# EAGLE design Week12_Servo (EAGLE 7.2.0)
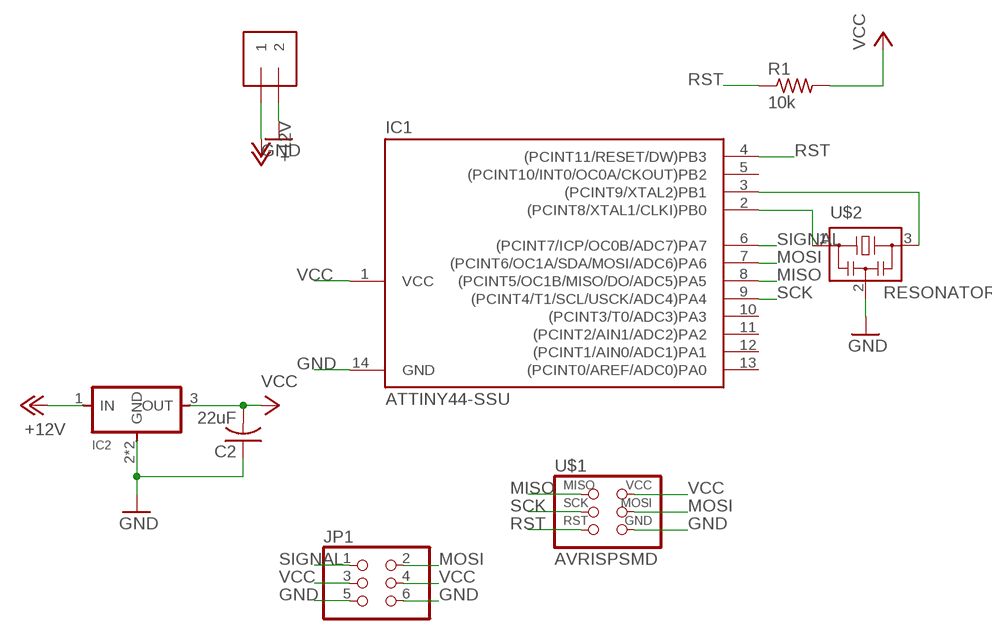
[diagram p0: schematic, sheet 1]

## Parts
C2  22uF  C-USC1206  [C1206]
IC1  ATTINY44-SSU  [SOIC14]
IC2  REGULATORSOT223  [SOT223]
J1  1X2-3.5MM  [3.5MMTERM]
JP1  PINHD-2X3-SMD  [2X03SMD]
R1  10k  RESISTOR1206  [1206]
U$1  AVRISPSMD  [2X03SMD]
U$2  RESONATOR  [EFOBM]

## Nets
+12V: IC2.1(IN) J1.1
GND: C2.1 IC1.14(GND) IC2.2(GND) IC2.4(GND) J1.2 JP1.5 JP1.6 U$1.6(GND) U$2.2
MISO: IC1.8((PCINT5/OC1B/MISO/DO/ADC5)PA5) U$1.1(MISO)
MOSI: IC1.7((PCINT6/OC1A/SDA/MOSI/ADC6)PA6) JP1.2 U$1.4(MOSI)
N$1: IC1.3((PCINT9/XTAL2)PB1) U$2.3
N$2: IC1.2((PCINT8/XTAL1/CLKI)PB0) U$2.1
RST: IC1.4((PCINT11/RESET/DW)PB3) R1.1 U$1.5(RST)
SCK: IC1.9((PCINT4/T1/SCL/USCK/ADC4)PA4) U$1.3(SCK)
SIGNAL: IC1.6((PCINT7/ICP/OC0B/ADC7)PA7) JP1.1
VCC: C2.2 IC1.1(VCC) IC2.3(OUT) JP1.3 JP1.4 R1.2 U$1.2(VCC)
Unconnected: IC1.5((PCINT10/INT0/OC0A/CKOUT)PB2) IC1.10((PCINT3/T0/ADC3)PA3) IC1.11((PCINT2/AIN1/ADC2)PA2) IC1.12((PCINT1/AIN0/ADC1)PA1) IC1.13((PCINT0/AREF/ADC0)PA0)

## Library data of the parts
C2 = 01_adafruit:C-US: CAPACITOR, American symbol
IC1 = 01_FAB_Hello:ATTINY44
IC2 = 01_fab:REGULATOR
J1 = 01_adafruit:1X2: 3.5mm Terminal block
JP1 = 01_FAB_Hello:PINHD-2X3-SMD: PIN HEADER
R1 = 01_FAB_Hello:RESISTOR
U$1 = 01_FAB_Hello:AVRISP
U$2 = 01_fab:RESONATOR

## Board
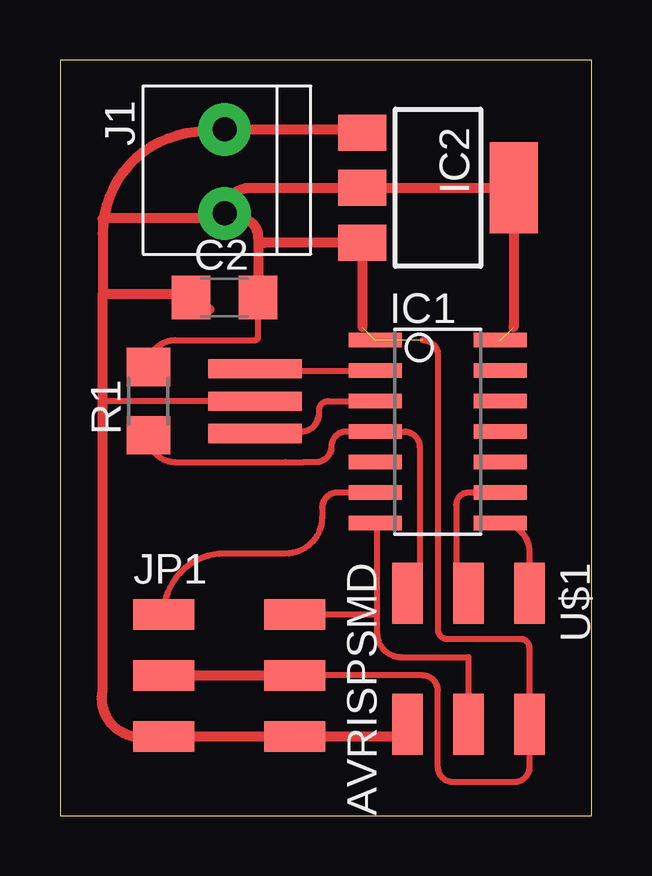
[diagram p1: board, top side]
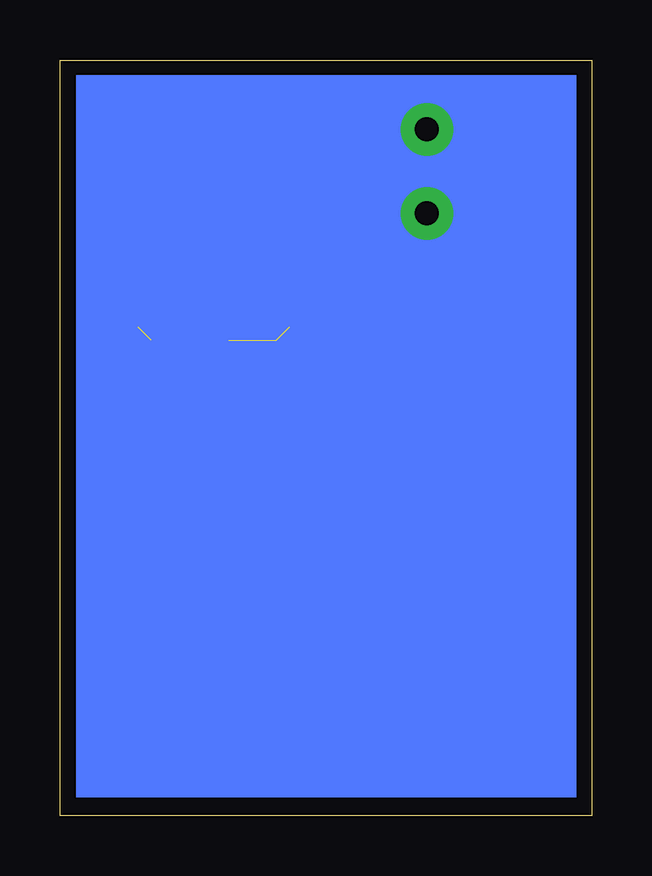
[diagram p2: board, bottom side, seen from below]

Size 22.15 x 31.49 mm. Coordinates in mm from the lower left corner, seen from the top.
Outline: 0,0 22.15,0 22.15,31.49 0,31.49 0,0
Copper layers (1*16): Top 0.035mm / dielectric 1.5mm / Bottom 0.035mm
Design rules "fabmodule": minimum track width 10mil, minimum drill 0.4mm, track to track 0.42mm, track to pad 0.42mm, pad to pad 0.42mm, via to via 0.42mm, smd to smd 0.42mm, copper to edge 40mil, drill to drill 0.8mm, minimum pad ring 10mil, minimum via ring 8mil, stop-mask expansion 4mil, vias tented up to drill 0mil, thermal gap 10mil

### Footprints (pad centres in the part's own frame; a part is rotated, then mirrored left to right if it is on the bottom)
C1206 = smd 1.6 x 1.8: 1 -1.4,0; 2 1.4,0
SOIC14 = smd 0.61 x 2.21: 1 -3.81,-2.603; 2 -2.54,-2.603; 3 -1.27,-2.603; 4 0,-2.603; 5 1.27,-2.603; 6 2.54,-2.603; 7 3.81,-2.603; 8 3.81,2.603; 9 2.54,2.603; 10 1.27,2.603; 11 0,2.603; 12 -1.27,2.603; 13 -2.54,2.603; 14 -3.81,2.603
SOT223 = smd 1.5 x 2: 1 -2.3,-3.15; 2 0,-3.15; 3 2.3,-3.15 | smd 3.8 x 2: 4 0,3.15
3.5MMTERM = drill 1 pad 2.184: 1 1.8,0; 2 -1.7,0
2X03SMD = smd 2.54 x 1.27: 1 -2.54,2.54; 2 2.92,2.54; 3 -2.54,0; 4 2.92,0; 5 -2.54,-2.54; 6 2.92,-2.54
1206 = smd 1.6 x 1.803: 1 -1.422,0; 2 1.422,0
EFOBM = smd 0.8 x 3.9: 1 -1.35,0; 2 0,0; 3 1.35,0

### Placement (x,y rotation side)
C2  6.86,21.59 0 top
IC1  15.75,16 270 top
IC2  15.75,26.16 270 top
J1  6.86,26.8 90 top
JP1  6.86,5.84 0 top
R1  3.68,17.27 90 top
U$1  17.02,6.73 270 top
U$2  8.13,17.27 270 top

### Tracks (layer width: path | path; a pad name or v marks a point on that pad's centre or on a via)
+12V
  Top 0.406: J1.1 12.6,28.6 IC2.1
GND  (1 unrouted)
  Top 0.254: U$2.2 1.78,17.27
  Top 0.406: U$1.6 14.48,3.56 arc-90 14.22,3.3 JP1.6 JP1.5 3.05,3.3 arc-90 1.78,5.21 1.78,17.27 1.78,21.72 | 18.9,20.36 IC2.4 IC2.2 7.92,26.16 arc90 J1.2 arc-90 6.65,24.89 1.78,24.89 1.78,24.26 | 6.22,21.08 C2.1 arc90 5.33,21.72 1.78,21.72 | 6.02,28.5 arc90 1.78,24.26 | 1.78,24.26 1.78,21.72
MISO
  Top 0.254: IC1.8 arc-90 19.56,10.98 U$1.1
MOSI
  Top 0.254: IC1.7 arc-90 13.21,12.13 13.21,8.38 | 13.21,8.38 13.21,7.62 arc90 14.22,6.6 17.02,6.6 U$1.4 | JP1.2 13.21,8.38
N$1
  Top 0.254: U$2.3 arc-90 8.21,16 10.03,16 arc90 10.79,16.76 10.79,16.89 arc-90 11.18,17.27 IC1.3
N$2
  Top 0.254: U$2.1 arc90 8.21,18.54 IC1.2
RST
  Top 0.254: U$1.5 arc90 14.86,9.65 arc90 14.99,9.78 14.99,15.37 arc90 14.35,16 IC1.4 11.94,16 arc90 11.3,15.37 arc-90 10.67,14.73 10.16,14.73 9.4,14.73 4.8,14.73 arc-90 R1.1
  Top 0.406: 14.86,10.03 14.73,10.03 arc90 14.48,9.78 U$1.5
SCK
  Top 0.254: IC1.9 17.02,13.46 arc90 16.51,12.95 16.51,9.78 arc90 U$1.3
SIGNAL
  Top 0.254: IC1.6 11.56,13.46 arc90 10.92,12.83 10.92,12.45 arc-90 9.4,10.92 6.86,10.92 arc90 JP1.1
VCC  (2 unrouted)
  Top 0.254: 15.11,19.81 arc-90 15.75,19.18 15.75,7.75 arc90 16.13,7.37 19.18,7.37 arc-90 19.56,6.98 U$1.2 19.56,2.03 arc-90 18.92,1.4 16.38,1.4 arc-90 15.75,2.03 15.75,5.21 arc90 15.11,5.84 JP1.4 | R1.2 arc-90 4.8,19.81 8.13,19.81 arc90 8.26,19.94 C2.2
  Top 0.406: JP1.3 JP1.4 | 8.26,24.12 C2.2 | 8.26,24.12 arc90 8.51,23.86 IC2.3 12.6,20.36 | 7.49,24.89 arc90 7.39,25 6.96,25 arc90 6.86,24.89 7.49,24.89 | 8.26,24.12 8.26,24.13 arc90 7.49,24.89
(copper drawn outside any net)
  shapes: Bottom area x1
